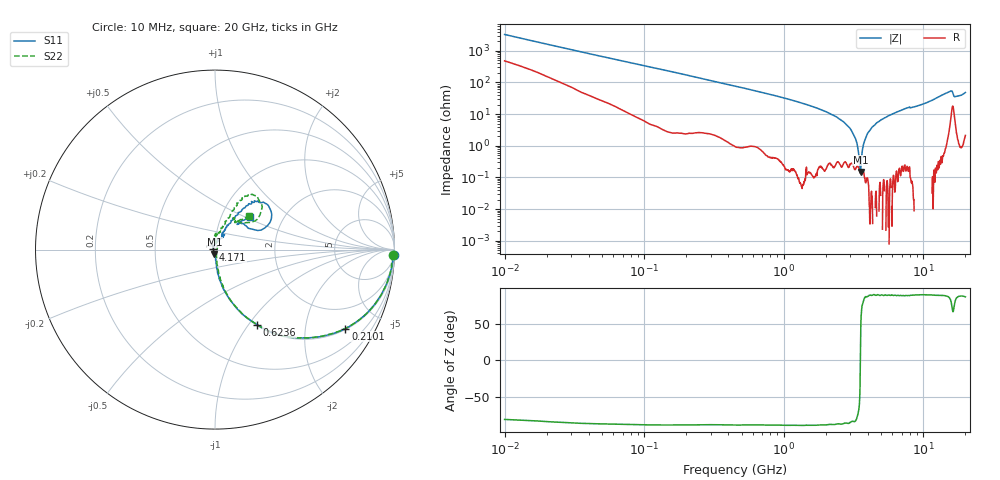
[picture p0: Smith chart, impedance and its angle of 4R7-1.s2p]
!Keysight Technologies,P5008B,MY61100088,A.16.20.02
!Date: Monday, May 27, 2024 16:20:09
!Correction: S11(C* 2-Port  )
!S21(C* 2-Port  )
!S12(C* 2-Port  )
!S22(C* 2-Port  )
!S2P File: Measurements: S11, S21, S12, S22:Log Frequency Sweep
# Hz S  dB  R 50
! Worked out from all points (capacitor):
!   1601 points, 10 MHz to 20 GHz, reference 50 ohm
!   read as one part in series: C = 4.91 pF near 10.39 MHz
!   lowest |Z| = 148 mohm at 3.549 GHz (marker M1)
!   series resonance near 3.537 GHz, so ESL is about 410 pH
!   S11 on the Smith chart (normalised r, x): 10 MHz: 6, -66; 210.1 MHz: 1.04, -3.28; 623.6 MHz: 1.01, -1.09; 4.171 GHz: 0.98, +0.00; 20 GHz: 1.37, +0.53
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1e7  -0.03 -1.7  -30.36 79.9  -30.38 80.0  -0.05 -1.7
3.555162e7  -0.10 -6.1  -19.38 80.8  -19.38 80.8  -0.10 -6.2
1.263918e8  -0.61 -20.3  -9.23 68.9  -9.25 68.9  -0.60 -20.3
2.101237e8  -1.42 -31.2  -5.78 58.0  -5.79 58.0  -1.42 -31.1
4.472136e8  -4.37 -52.3  -2.07 37.0  -2.08 37.0  -4.35 -52.3
6.236416e8  -6.41 -60.8  -1.19 28.1  -1.20 28.1  -6.43 -60.9
1.589917e9  -14.93 -80.6  -0.14 9.5  -0.15 9.5  -14.85 -79.1
2.681144e9  -22.73 -85.4  -0.02 2.3  -0.03 2.3  -22.64 -81.4
3.196366e9  -27.69 -90.1  -0.00 0.0  -0.01 0.0  -28.13 -78.3
3.548507e9  -31.93 -98.2  0.00 -1.4  -0.00 -1.4  -33.32 -66.8
3.883698e9  -38.29 -126.2  0.01 -2.6  -0.00 -2.6  -38.84 -21.3
4.170543e9  -39.91 175.3  0.01 -3.5  0.00 -3.5  -37.48 22.1
4.786562e9  -33.44 108.3  0.01 -5.4  0.00 -5.5  -32.34 60.3
5.652411e9  -27.32 79.3  0.01 -7.8  -0.00 -7.8  -27.45 82.1
7.660815e9  -20.68 58.2  -0.01 -13.0  -0.01 -13.0  -21.05 87.3
8.344716e9  -21.76 58.2  0.01 -14.4  0.00 -14.4  -21.88 86.3
9.854205e9  -20.25 66.7  0.01 -18.2  -0.01 -18.2  -20.26 75.6
1.518335e10  -8.88 47.1  -0.73 -33.6  -0.73 -33.6  -8.88 56.9
1.592205e10  -8.44 34.3  -1.48 -34.0  -1.49 -34.1  -8.82 44.3
1.717946e10  -13.33 42.4  -0.38 -29.6  -0.39 -29.6  -13.72 59.6
1.862442e10  -14.38 47.6  -0.18 -35.6  -0.19 -35.6  -14.40 53.2
2e10  -11.49 42.6  -0.44 -40.8  -0.44 -40.8  -11.38 44.7
